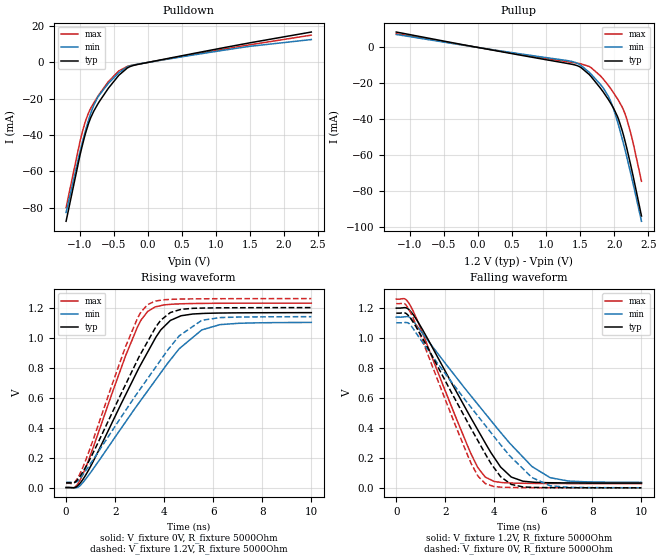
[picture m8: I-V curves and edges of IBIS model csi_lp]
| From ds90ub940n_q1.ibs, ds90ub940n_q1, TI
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|   Model
[Model]   csi_lp
Model_type   Output
Polarity   Non-Inverting
Vmeas = 0.6
Vref = 0
Cref = 1pF
Rref = 100000
|   typ   min   max
C_comp   0.31pF   0.27pF   0.33pF
[Voltage Range]   1.2   1.14   1.26
[Temperature Range]   27   105   -40
[Pullup Reference]   1.2   1.14   1.26
[Pulldown Reference]   0   0   0
[Power Clamp Reference]   1.2   1.14   1.26
[GND Clamp Reference]   0   0   0
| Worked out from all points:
|   slope of the pulldown table from 0 to 0.18 V, typ, clamps not added: 135 ohm
|   slope of the pullup table from 0 to 0.18 V, typ, clamps not added: 144 ohm
|   falling waveform, V_fixture 1.2V, R_fixture 5000Ohm: 20-80 % time 2.37ns typ, 3.28ns min, 1.8ns max; typ from 1.2 V to 0.032 V
|   rising waveform, V_fixture 0V, R_fixture 5000Ohm: 20-80 % time 2.14ns typ, 2.88ns min, 1.63ns max; typ from 0 V to 1.17 V
|   rising waveform, V_fixture 1.2V, R_fixture 5000Ohm: 20-80 % time 2.1ns typ, 2.77ns min, 1.61ns max; typ from 0.031 V to 1.2 V
|   falling waveform, V_fixture 0V, R_fixture 5000Ohm: 20-80 % time 2.32ns typ, 3.13ns min, 1.77ns max; typ from 1.17 V to 0 V
[Pulldown]
|   Voltage   I(typ)   I(min)   I(max)
-1.2V     -87.39mA   -82.55mA   -79.88mA
-998.4mV  -51.49mA   -49.45mA   -43.9mA
-930mV    -41.07mA   -39.48mA   -34.1mA
-868.8mV  -33.44mA   -31.5mA    -27.64mA
-793.2mV  -26.81mA   -23.56mA   -22.26mA
-714mV    -21.63mA   -18.01mA   -17.53mA
-573.6mV  -13.92mA   -11.35mA   -10.32mA
-426mV    -7.084mA   -5.673mA   -4.716mA
-300mV    -3.034mA   -2.46mA    -2.172mA
-145.2mV  -1.092mA   -921.7uA   -971.1uA
1.262V    9.144mA    7.554mA    8.241mA
2.4V      16.72mA    12.58mA    15.02mA
[Pullup]
|   Voltage   I(typ)   I(min)   I(max)
-1.2V     8.607mA    7.249mA    7.676mA
1.331V    -9.037mA   -7.45mA    -8.066mA
1.511V    -11.16mA   -9.989mA   -9.14mA
1.658V    -16.17mA   -14.83mA   -11.22mA
1.835V    -24.65mA   -22.42mA   -17.43mA
1.914V    -29.07mA   -27.25mA   -21.18mA
1.968V    -32.43mA   -32.05mA   -24.08mA
2.065V    -40.27mA   -43.72mA   -29.77mA
2.13V     -48.18mA   -52.91mA   -34.39mA
2.184V    -56.19mA   -61.1mA    -39.89mA
2.278V    -71.84mA   -76.14mA   -53.34mA
2.4V      -94.06mA   -97mA      -74.69mA
[Ramp]
R_load = 5000
|   typ   min   max
dV/dt_r   0.699587/2.14058e-09   0.660502/2.88285e-09   0.737673/1.63315e-09
dV/dt_f   0.700893/2.37369e-09   0.661959/3.27729e-09   0.738824/1.80343e-09
[Falling Waveform]
V_fixture = 1.2V
V_fixture_min = 1.14V
V_fixture_max = 1.26V
R_fixture = 5000Ohm
C_fixture = 0F
|   Time   V(typ)   V(min)   V(max)
0s        1.2V       1.14V      1.26V
396.2ps   1.202V     1.143V     1.257V
668.8ps   1.161V     1.119V     1.187V
3.052ns   464.9mV    612.8mV    225.8mV
3.63ns    299.1mV    495.9mV    71.8mV
4.253ns   139.2mV    370.7mV    36.74mV
4.688ns   72.37mV    287.7mV    32.26mV
5.533ns   38.67mV    142.5mV    29.92mV
6.276ns   34.17mV    67.91mV    29.2mV
10ns      31.79mV    36.65mV    28.47mV
[Rising Waveform]
V_fixture = 0V
V_fixture_min = 0V
V_fixture_max = 0V
R_fixture = 5000Ohm
C_fixture = 0F
|   Time   V(typ)   V(min)   V(max)
0s        18.58uV    27.85uV    28.83uV
335.5ps   -1.009mV   -1.085mV   210.3uV
668.8ps   50.29mV    30.28mV    82.82mV
2.426ns   617.8mV    437.2mV    878.1mV
2.915ns   779.4mV    551.9mV    1.072V
3.325ns   902.5mV    644.1mV    1.174V
4.253ns   1.114V     851.4mV    1.221V
5.533ns   1.16V      1.051V     1.228V
7.024ns   1.165V     1.095V     1.229V
10ns      1.166V     1.101V     1.229V
[Rising Waveform]
V_fixture = 1.2V
V_fixture_min = 1.14V
V_fixture_max = 1.26V
R_fixture = 5000Ohm
C_fixture = 0F
|   Time   V(typ)   V(min)   V(max)
0s        31.47mV    35.35mV    28.34mV
335.5ps   32.9mV     34.79mV    32.92mV
589.4ps   80.05mV    64.18mV    100.1mV
2.426ns   686.9mV    513.3mV    939.7mV
2.915ns   851.8mV    631.9mV    1.13V
3.325ns   973.5mV    726.7mV    1.22V
3.862ns   1.116V     851.1mV    1.249V
4.253ns   1.167V     938.8mV    1.254V
5.533ns   1.196V     1.115V     1.258V
10ns      1.2V       1.139V     1.26V
[Falling Waveform]
|Gnd
V_fixture = 0V
V_fixture_min = 0V
V_fixture_max = 0V
R_fixture = 5000Ohm
C_fixture = 0F
|   Time   V(typ)   V(min)   V(max)
0s        1.166V     1.102V     1.23V
335.5ps   1.168V     1.104V     1.23V
589.4ps   1.13V      1.086V     1.167V
3.052ns   395.5mV    536.8mV    163.5mV
3.63ns    227.1mV    416.7mV    28.49mV
4.253ns   74.72mV    288.1mV    4.98mV
4.688ns   23.14mV    204.3mV    2.45mV
5.533ns   3.488mV    68.84mV    1.111mV
6.276ns   1.481mV    13.75mV    663.1uV
10ns      232.3uV    677.9uV    138.9uV
